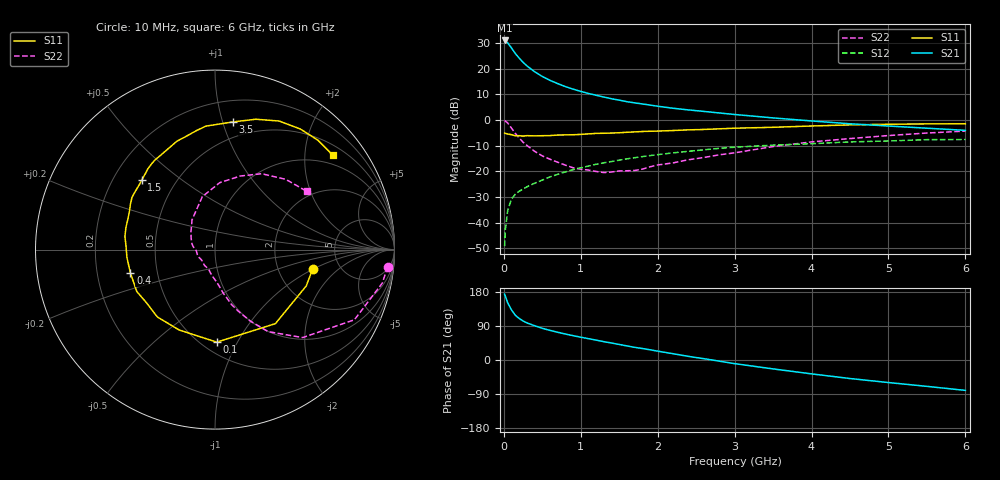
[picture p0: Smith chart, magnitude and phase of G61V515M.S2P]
! SIEMENS Small Signal Semiconductors
! BFG193
! Si NPN RF Bipolar Junction Transistor in SOT223
! VCE = 1.5 V  IC = 15 mA
! Common Emitter S-Parameters:  August  1996
# GHz  S  MA  R  50
!  f  S11  S21  S12  S22
! GHz  MAG  ANG  MAG  ANG  MAG  ANG  MAG  ANG
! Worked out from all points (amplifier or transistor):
!   36 points, 10 MHz to 6 GHz, reference 50 ohm
!   highest |S21| = 30.9 dB at 10 MHz (marker M1)
!   |S21| within 3 dB of that: start of sweep to 101.5 MHz
!   unconditionally stable (mu >= 1): 732.5 MHz to 2.747 GHz
!   at 250 MHz: K = 0.68, MSG = 24.7 dB, |S12| = -26.9 dB
!   at 1.4 GHz: K = 1.07, MAG = 10.6 dB, |S12| = -16.2 dB
!   at 6 GHz: K = 0.93, MSG = 1.8 dB, |S12| = -7.6 dB
!   S11 on the Smith chart (normalised r, x): 10 MHz: 3.16, -0.98; 100 MHz: 0.59, -0.83; 400 MHz: 0.35, -0.12; 1.5 GHz: 0.32, +0.36; 3.5 GHz: 0.37, +1.08; 6 GHz: 0.74, +2.66
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0.01  0.5549 -11.1  35.11 173.6  0.0035 88.6  0.9661 -5.7
0.02  0.5473 -21.7  34.62 168.2  0.0074 84.0  0.9509 -11.3
0.05  0.5323 -50.8  31.51 151.0  0.0172 70.6  0.8697 -26.7
0.1  0.5157 -88.9  25.04 131.9  0.029 59.9  0.692 -45.1
0.15  0.4904 -114.0  19.5 118.0  0.036 53.5  0.5452 -57.0
0.2  0.494 -130.5  15.89 109.6  0.0411 52.7  0.4456 -63.6
0.25  0.4833 -142.7  13.2 102.9  0.0452 51.7  0.368 -69.2
0.3  0.4944 -151.8  11.26 97.9  0.05 52.5  0.3189 -73.3
0.4  0.4889 -164.4  8.661 90.4  0.0586 53.1  0.2454 -79.4
0.5  0.4927 -174.8  6.994 83.6  0.0676 53.6  0.1993 -84.2
0.6  0.4959 178.0  5.889 78.2  0.0779 54.4  0.1717 -89.1
0.7  0.5072 171.7  5.082 73.2  0.0873 54.0  0.1503 -95.0
0.9  0.5144 160.5  3.971 64.2  0.1078 52.1  0.1171 -106.8
1.1  0.5349 151.8  3.27 56.3  0.1267 50.0  0.1057 -123.2
1.5  0.5628 136.5  2.425 41.0  0.1647 43.1  0.1018 -157.5
1.7  0.5848 129.9  2.145 33.5  0.1839 39.4  0.1038 -175.1
2.2  0.6215 114.3  1.685 16.6  0.2287 28.6  0.1459 155.5
3  0.6898 94.2  1.275 -9.6  0.2948 10.9  0.2289 119.7
3.5  0.7184 82.0  1.094 -23.5  0.3229 -1.8  0.3032 103.5
4.5  0.8004 63.5  0.841 -48.9  0.373 -21.3  0.4336 71.0
5.5  0.8366 46.8  0.69 -69.6  0.4128 -44.1  0.5555 44.8
6  0.8411 38.8  0.626 -80.2  0.4159 -57.1  0.6063 32.3
